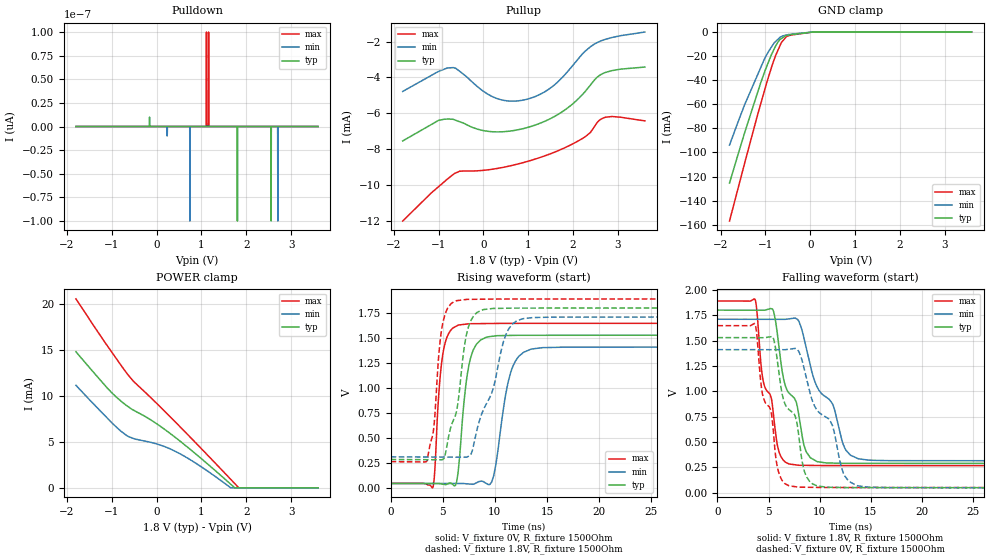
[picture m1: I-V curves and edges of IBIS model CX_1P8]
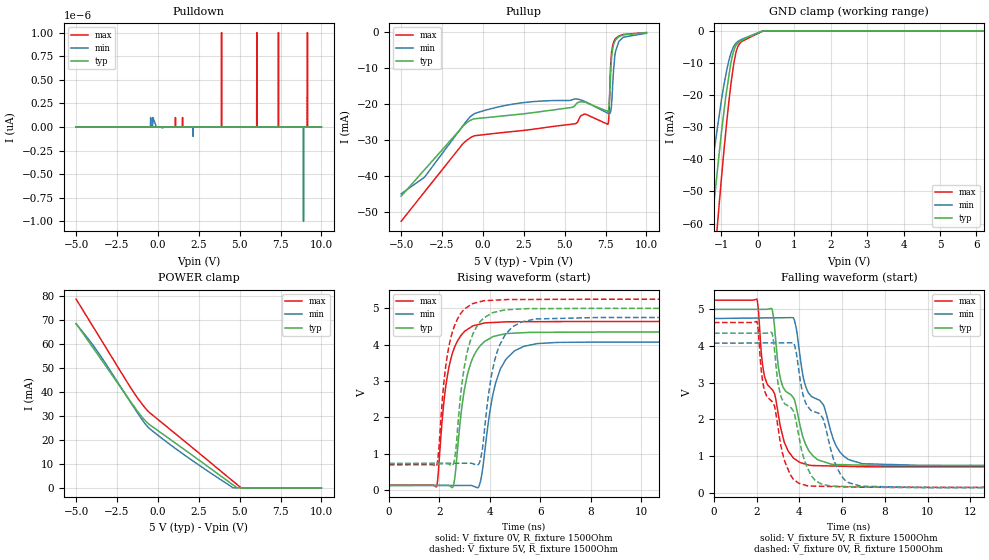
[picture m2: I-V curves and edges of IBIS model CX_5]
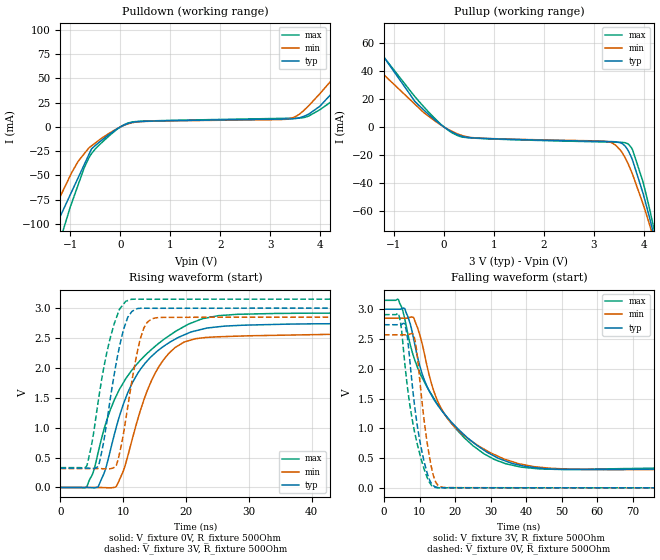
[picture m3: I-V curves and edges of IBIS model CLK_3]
| Texas Instruments Incorporated
| Smart Card Interface IC for 1 User Card + 3 SAMs
| Marketing part#   Voltage Range   Package-type   #pins/pkg drawing
| TCA5013ZAH   1.65V - 5.5V   nFBGA   48-pin ZAH
[IBIS Ver]   4.1
[File name]   tca5013.ibs
[File Rev]   1.0
[Date]   07/24/2014
[Source]   Model built from spectre simulations at:
   Texas Instruments Incorporated.
   Analog-eLab, HPA
   12500 TI Blvd
   Dallas, TX -75243
   For Support e-mail: elab_ibis@list.ti.com
[Notes]   Revision History
   Rev 1.0: 07/24/2014
   - Pullup and Pulldown is non-monotonic for many buffers
   - ccomp values are based on PVT settings:
   MIN: Low Voltage, High Temperature, Weak Process
   TYP: Nominal Voltage, Nominal Temperature, Nominal Process
   MAX: High Voltage, Low Temperature, Fast Process
   - C_comp although listed in numerical order of value are obtained from varying PVT conditions.
   For PVT conditions for each specific value, refer to the buffer description under respective [Model].
   IBIS model user is responsible for using appropriate C_comp to simulate for Signal Integrity.
[Disclaimer]  This model is designed as an aid for customers of Texas Instruments
 TI and its licensors and suppliers make no warranties, either expressed
 or implied, with respect to this  model, including the warranties of
 merchantability or fitness for a particular purpose.
 The model is provided solely on an "as is" basis. The entire risk as to
 its quality and performance is with the customer.
[Copyright] (C)Copyright 2014 Texas Instruments Incorporated.
   All rights reserved.
[Component]   TCA5013ZAH
[Manufacturer]  Texas Instruments Incorporated
[Package]   |48-pin nFBGA ZAH package
|   typ   min   max
R_pkg   0.005   0.005   0.005
L_pkg   0.2n   0.2n   0.2n
C_pkg   0.6p   0.6p   0.6p
[Pin]   signal_name   model_name   R_pin   L_pin   C_pin
A1   PRES   PRES   0.005   0.2nH   0.6pF
A2   GPIO4   GPIO   0.005   0.2nH   0.6pF
A4   GPIO3   GPIO   0.005   0.2nH   0.6pF
A5   GPIO2   GPIO   0.005   0.2nH   0.6pF
A6   GPIO1   GPIO   0.005   0.2nH   0.6pF
A8   VUP   NC   0.005   0.2nH   0.6pF
A9   LX   NC   0.005   0.2nH   0.6pF
B1   C8   CX   0.005   0.2nH   0.6pF
B2   A0   SCL   0.005   0.2nH   0.6pF
B3   INT   INT   0.005   0.2nH   0.6pF
B4   SHDN   PRES   0.005   0.2nH   0.6pF
B5   SCL   SCL   0.005   0.2nH   0.6pF
B6   SDA   SDA   0.005   0.2nH   0.6pF
B7   LDOCAP   NC   0.005   0.2nH   0.6pF
B8   TST4   NC   0.005   0.2nH   0.6pF
B9   GNDP   GND   0.005   0.2nH   0.6pF
C2   C4   CX   0.005   0.2nH   0.6pF
C8   VDD   POWER   0.005   0.2nH   0.6pF
D1   CLKUC   CLK   0.005   0.2nH   0.6pF
D2   TST3   NC   0.005   0.2nH   0.6pF
D8   GND   GND   0.005   0.2nH   0.6pF
D9   CLKIN1   CLKIN   0.005   0.2nH   0.6pF
E1   GNDUC   GND   0.005   0.2nH   0.6pF
E2   IOUC   IO   0.005   0.2nH   0.6pF
E8   IOMC1   IOMC   0.005   0.2nH   0.6pF
E9   GND   GND   0.005   0.2nH   0.6pF
F1   RSTUC   RST   0.005   0.2nH   0.6pF
F2   VCCUC   POWER   0.005   0.2nH   0.6pF
F8   IOMC2   IOMC   0.005   0.2nH   0.6pF
F9   CLKIN2   CLKIN   0.005   0.2nH   0.6pF
G2   TST2   NC   0.005   0.2nH   0.6pF
G8   VDDI   POWER   0.005   0.2nH   0.6pF
H1   RSTS3   RST   0.005   0.2nH   0.6pF
H2   IOS3   IO   0.005   0.2nH   0.6pF
H3   GNDS   GND   0.005   0.2nH   0.6pF
H4   TST1   NC   0.005   0.2nH   0.6pF
H5   IOS2   IO   0.005   0.2nH   0.6pF
H6   GNDS   GND   0.005   0.2nH   0.6pF
H7   GNDS   GND   0.005   0.2nH   0.6pF
H8   IOS1   IO   0.005   0.2nH   0.6pF
H9   VCCS1   POWER   0.005   0.2nH   0.6pF
J1   CLKS3   CLK   0.005   0.2nH   0.6pF
J2   VCCS3   POWER   0.005   0.2nH   0.6pF
J4   RSTS2   RST   0.005   0.2nH   0.6pF
J5   CLKS2   CLK   0.005   0.2nH   0.6pF
J6   VCCS2   POWER   0.005   0.2nH   0.6pF
J8   RSTS1   RST   0.005   0.2nH   0.6pF
J9   CLKS1   CLK   0.005   0.2nH   0.6pF
[Model Selector] CLK
CLK_1P8   CLK OUTPUT 1.8V
CLK_3   CLK OUTPUT 3V
CLK_5   CLK OUTPUT 5V
[Model Selector] CLKIN
CLKIN_1P8   CLKIN INPUT 1.8V
CLKIN_2P5   CLKIN INPUT 2.5V
CLKIN_3P3   CLKIN INPUT 3.3V
[Model Selector] RST
RST_1P8   RST OUTPUT 1.8V
RST_3   RST OUTPUT 3V
RST_5   RST OUTPUT 5V
[Model Selector] IO
IO_1P8   IO OUTPUT 1.8V
IO_3   IO OUTPUT 3V
IO_5   IO OUTPUT 5V
[Model Selector] IOMC
IOMC_1P8   IOMC OUTPUT 1.8V
IOMC_3   IOMC OUTPUT 3V
IOMC_5   IOMC OUTPUT 5V
[Model Selector] CX
CX_1P8   CX OUTPUT 1.8V
CX_3   CX OUTPUT 3V
CX_5   CX OUTPUT 5V
[Model Selector] SDA
SDA_1P8   SDA OPEN DRAIN I/O 1.8V
SDA_2P5   SDA OPEN DRAIN I/O 2.5V
SDA_3P3   SDA OPEN DRAIN I/O 3.3V
[Model Selector] GPIO
GPIO_1P8   GPIO OPEN DRAIN I/O 1.8V
GPIO_2P5   GPIO OPEN DRAIN I/O 2.5V
GPIO_3P3   GPIO OPEN DRAIN I/O 3.3V
[Model Selector] INT
INT_1P8   INT OPEN DRAIN OUTPUT 1.8V
INT_2P5   INT OPEN DRAIN OUTPUT 2.5V
INT_3P3   INT OPEN DRAIN OUTPUT 3.3V
[Model Selector] SCL
SCL_1P8   SCL INPUT 1.8V
SCL_2P5   SCL INPUT 2.5V
SCL_3P3   SCL INPUT 3.3V
[Model Selector] PRES
PRES_1P8   PRES INPUT 1.8V
PRES_2P5   PRES INPUT 2.5V
PRES_3P3   PRES INPUT 3.3V
| Models and submodels in the file (33): CX_1P8 (I/O), CX_3 (I/O), CX_5 (I/O), CLK_1P8 (Output), CLK_3 (Output), CLK_5 (Output), CLKIN_1P8 (Input), CLKIN_2P5 (Input), CLKIN_3P3 (Input), GPIO_1P8 (I/O_open_drain), GPIO_2P5 (I/O_open_drain), GPIO_3P3 (I/O_open_drain), INT_1P8 (Open_drain), INT_3P3 (Open_drain), INT_2P5 (Open_drain), IO_1P8 (I/O), IO_3 (I/O), IO_5 (I/O), IOMC_1P8 (I/O), IOMC_3 (I/O), IOMC_5 (I/O), PRES_1P8 (Input), PRES_2P5 (Input), PRES_3P3 (Input), RST_1P8 (Output), RST_3 (Output), RST_5 (Output), SCL_1P8 (Input), SCL_2P5 (Input), SCL_3P3 (Input), SDA_1P8 (I/O_open_drain), SDA_2P5 (I/O_open_drain), SDA_3P3 (I/O_open_drain)
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|   Model CX
[Model]   CX_1P8
Model_type   I/O
Polarity   Non-Inverting
Enable   Active-Low
Vinl = 0.72
Vinh = 1.08
Vmeas = 0.9
Vref = 1.8
Cref = 1pF
Rref = 1500
|   typ   min   max
C_comp   0.597p   0.445p   0.907p
|C_comp (ON state)   0.597p   0.445p   0.907p
|C_comp (OFF state)   0.592p   0.445p   0.907p
[Model spec]
|subparameter
Vinl   0.72   0.684   0.756
Vinh   1.08   1.026   1.134
[Voltage Range]   1.8   1.71   1.89
[Temperature Range]   27   125   -40
[Pullup Reference]   1.8   1.71   1.89
[Pulldown Reference]   0   0   0
[Power Clamp Reference]   1.8   1.71   1.89
[GND Clamp Reference]   0   0   0
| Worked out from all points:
|   slope of the pullup table from 0 to 0.27 V, typ, clamps not added: 3.81 kohm
|   GND clamp passes 1 mA (typ) near -0.17 V on its own axis
|   falling waveform, V_fixture 1.8V, R_fixture 1500Ohm: 20-80 % time 2.29ns typ, 3.31ns min, 1.65ns max; typ from 1.8 V to 0.289 V
|   rising waveform, V_fixture 0V, R_fixture 1500Ohm: 20-80 % time 876ps typ, 1.26ns min, 656ps max; typ from 0.05 V to 1.53 V
|   rising waveform, V_fixture 1.8V, R_fixture 1500Ohm: 20-80 % time 1.49ns typ, 2.43ns min, 743ps max; typ from 0.289 V to 1.8 V
|   falling waveform, V_fixture 0V, R_fixture 1500Ohm: 20-80 % time 2.27ns typ, 3.28ns min, 1.64ns max; typ from 1.53 V to 0.05 V
[Pulldown]
|   Voltage   I(typ)   I(min)   I(max)
-1.8V     0A         0A         0A
738mV     0A         0A         0A
743.4mV   0A         -100fA     0A
1.111V    0A         0A         100fA
1.802V    -100fA     0A         0A
1.807V    0A         0A         0A
2.547V    0A         0A         0A
2.552V    -100fA     0A         0A
2.698V    0A         0A         0A
2.704V    0A         -100fA     0A
2.709V    0A         0A         0A
3.6V      0A         0A         0A
[GND Clamp]
|   Voltage   I(typ)   I(min)   I(max)
-1.8V     -125.5mA   -93.9mA    -156.9mA
-1.465V   -83.92mA   -60.61mA   -109.3mA
-1.106V   -42.36mA   -29.69mA   -59.83mA
-995.4mV  -30.89mA   -20.6mA    -45.41mA
-844.2mV  -17.17mA   -11.26mA   -27.11mA
-774mV    -11.72mA   -7.931mA   -19.72mA
-725.4mV  -8.655mA   -6.195mA   -15.61mA
-644.4mV  -5.413mA   -3.754mA   -8.753mA
-531mV    -2.861mA   -2.501mA   -3.795mA
-423mV    -2.124mA   -1.831mA   -2.525mA
57.6mV    -11.54uA   -2.781uA   -1.994uA
3.6V      0A         0A         0A
[Pullup]
|   Voltage   I(typ)   I(min)   I(max)
-1.8V     -7.545mA   -4.782mA   -12.02mA
-995.4mV  -6.392mA   -3.659mA   -10.09mA
-671.4mV  -6.343mA   -3.451mA   -9.417mA
235.8mV   -7.037mA   -5.113mA   -9.112mA
565.2mV   -7.005mA   -5.317mA   -8.956mA
937.8mV   -6.827mA   -5.24mA    -8.722mA
1.397V    -6.417mA   -4.758mA   -8.355mA
1.796V    -5.852mA   -3.901mA   -7.948mA
2.266V    -4.796mA   -2.542mA   -7.32mA
2.525V    -4.014mA   -2.068mA   -6.556mA
2.698V    -3.745mA   -1.89mA    -6.242mA
3.6V      -3.421mA   -1.466mA   -6.428mA
[POWER Clamp]
|   Voltage   I(typ)   I(min)   I(max)
-1.8V     14.79mA    11.15mA    20.54mA
-1.106V   10.88mA    7.607mA    15.49mA
-806.4mV  9.478mA    6.196mA    13.41mA
-671.4mV  8.948mA    5.697mA    12.5mA
-487.8mV  8.37mA     5.314mA    11.45mA
9mV       6.94mA     4.761mA    9.145mA
370.8mV   5.655mA    4.077mA    7.389mA
916.2mV   3.506mA    2.542mA    4.669mA
1.651V    400.1uA    3.806uA    933uA
1.742V    472.3nA    0A         461.4uA
1.829V    0A         0A         16.54uA
3.6V      0A         0A         0A
[Ramp]
R_load = 1500
|   typ   min   max
dV/dt_r   0.887602/8.76301e-10   0.816767/1.2525e-09   0.957567/6.56016e-10
dV/dt_f   0.906661/2.28507e-09   0.836809/3.30284e-09   0.973581/1.65071e-09
[Falling Waveform]
V_fixture = 1.8V
V_fixture_min = 1.71V
V_fixture_max = 1.89V
R_fixture = 1500Ohm
C_fixture = 0F
|   Time   V(typ)   V(min)   V(max)
0s        1.8V       1.71V      1.89V
3.691ns   1.799V     1.71V      1.903V
4.406ns   1.799V     1.71V      1.144V
5.447ns   1.8V       1.709V     800.5mV
6.032ns   1.43V      1.709V     402.2mV
7.004ns   983.1mV    1.714V     285mV
7.984ns   752.5mV    1.687V     271.8mV
9.087ns   346.5mV    1.257V     270.5mV
13.75ns   290.7mV    337.8mV    268.7mV
49.9ns    288.9mV    315.3mV    267.4mV
[Rising Waveform]
V_fixture = 0V
V_fixture_min = 0V
V_fixture_max = 0V
R_fixture = 1500Ohm
C_fixture = 0F
|   Time   V(typ)   V(min)   V(max)
0s        49.9mV     49.46mV    51.37mV
4.08ns    50.23mV    49.68mV    18.4mV
4.995ns   43.34mV    49.73mV    1.33V
6.487ns   171.8mV    49.81mV    1.628V
7.524ns   1.234V     44.82mV    1.642V
9.209ns   1.509V     48.67mV    1.644V
9.895ns   1.519V     129.5mV    1.645V
11.51ns   1.526V     1.154V     1.646V
13.44ns   1.527V     1.387V     1.646V
49.9ns    1.529V     1.411V     1.647V
[Rising Waveform]
V_fixture = 1.8V
V_fixture_min = 1.71V
V_fixture_max = 1.89V
R_fixture = 1500Ohm
C_fixture = 0F
|   Time   V(typ)   V(min)   V(max)
0s        288.9mV    315.3mV    267.3mV
3.498ns   287mV      313.7mV    277.8mV
4.132ns   286.6mV    313.5mV    596.9mV
4.944ns   287.8mV    313.1mV    1.616V
6.301ns   760.3mV    312.5mV    1.871V
7.175ns   1.479V     312.1mV    1.883V
7.956ns   1.719V     429.7mV    1.886V
11.04ns   1.796V     1.527V     1.888V
12.58ns   1.798V     1.689V     1.888V
49.9ns    1.8V       1.71V      1.89V
[Falling Waveform]
|Gnd
V_fixture = 0V
V_fixture_min = 0V
V_fixture_max = 0V
R_fixture = 1500Ohm
C_fixture = 0F
|   Time   V(typ)   V(min)   V(max)
0s        1.529V     1.411V     1.647V
3.691ns   1.528V     1.41V      1.661V
4.406ns   1.528V     1.41V      973.8mV
5.447ns   1.53V      1.41V      637.3mV
5.956ns   1.232V     1.41V      214.7mV
7.004ns   820mV      1.415V     69.52mV
7.984ns   543.2mV    1.389V     56.13mV
9.019ns   113.7mV    1.001V     54.77mV
13.63ns   51.62mV    72.17mV    52.81mV
49.9ns    49.9mV     49.46mV    51.37mV
[Model]   CX_5
Model_type   I/O
Polarity   Non-Inverting
Enable   Active-Low
Vinl = 2
Vinh = 3
Vmeas = 2.5
Vref = 5
Cref = 1pF
Rref = 1500
|   typ   min   max
|   typ   min   max
C_comp   0.937p   0.723p   1.081p
|C_comp (ON state)   0.950p   0.730p   1.090p
|C_comp (OFF state)   0.937p   0.723p   1.081p
[Model spec]
|subparameter
Vinl   2.0   1.9   2.1
Vinh   3.0   2.85   3.15
[Voltage Range]   5   4.75   5.25
[Temperature Range]   27   125   -40
[Pullup Reference]   5   4.75   5.25
[Pulldown Reference]   0   0   0
[Power Clamp Reference]   5   4.75   5.25
[GND Clamp Reference]   0   0   0
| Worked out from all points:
|   GND clamp passes 1 mA (typ) near -0.05 V on its own axis
|   falling waveform, V_fixture 5V, R_fixture 1500Ohm: 20-80 % time 1.24ns typ, 1.56ns min, 1.04ns max; typ from 5 V to 0.725 V
|   rising waveform, V_fixture 0V, R_fixture 1500Ohm: 20-80 % time 550ps typ, 617ps min, 493ps max; typ from 0.132 V to 4.35 V
|   rising waveform, V_fixture 5V, R_fixture 1500Ohm: 20-80 % time 539ps typ, 596ps min, 486ps max; typ from 0.725 V to 5 V
|   falling waveform, V_fixture 0V, R_fixture 1500Ohm: 20-80 % time 1.29ns typ, 1.61ns min, 1.07ns max; typ from 4.35 V to 0.132 V
[Pulldown]
|   Voltage   I(typ)   I(min)   I(max)
-5V       0A         0A         0A
3.88V     0A         0A         0A
3.895V    0A         0A         1pA
3.91V     0A         0A         0A
6.04V     0A         0A         0A
6.055V    0A         0A         1pA
6.07V     0A         0A         0A
7.375V    0A         0A         1pA
8.89V     0A         0A         0A
8.905V    0A         -1pA       0A
9.145V    0A         0A         1pA
10V       0A         0A         0A
[GND Clamp]
|   Voltage   I(typ)   I(min)   I(max)
-5V       -2.369A    -1.94A     -2.673A
-2.405V   -203.9mA   -160.8mA   -244.3mA
-1.205V   -54.28mA   -38.24mA   -73.88mA
-995mV    -31.76mA   -21.64mA   -46.02mA
-875mV    -20.5mA    -13.85mA   -31.48mA
-725mV    -9.458mA   -6.709mA   -15.86mA
-650mV    -6.128mA   -4.72mA    -9.891mA
-590mV    -4.508mA   -3.781mA   -6.49mA
-545mV    -3.908mA   -3.328mA   -4.894mA
-455mV    -3.039mA   -2.739mA   -3.493mA
145mV     -91.73uA   -1.815uA   -57.07uA
10V       0A         0A         0A
[Pullup]
|   Voltage   I(typ)   I(min)   I(max)
-5V       -45.57mA   -44.92mA   -52.52mA
-3.569V   -38.25mA   -40.32mA   -44.39mA
-500mV    -24.14mA   -22.71mA   -28.84mA
5.68V     -20.21mA   -18.66mA   -25.48mA
6.25V     -19.59mA   -19.38mA   -22.86mA
7.645V    -22.14mA   -22.64mA   -25.7mA
7.705V    -20.96mA   -22.74mA   -23.32mA
7.84V     -9.039mA   -21.39mA   -7.208mA
7.99V     -3.646mA   -10.63mA   -2.972mA
8.11V     -2.346mA   -5.507mA   -1.961mA
8.32V     -1.416mA   -2.689mA   -1.214mA
10V       -326.4uA   -476.2uA   -291.8uA
[POWER Clamp]
|   Voltage   I(typ)   I(min)   I(max)
-5V       68.6mA     68.49mA    78.81mA
-4.205V   60.85mA    61.75mA    69.99mA
-3.569V   54.65mA    55.74mA    62.94mA
-1.415V   33.6mA     33.08mA    39.2mA
-995mV    29.76mA    28.81mA    35.26mA
-605mV    26.96mA    25.4mA     32.05mA
265mV     22.63mA    20.58mA    27.1mA
1.6V      16.09mA    13.84mA    19.65mA
4.6V      1.234mA    20.62uA    2.752mA
4.84V     50.39uA    0A         1.415mA
5.08V     0A         0A         81.65uA
10V       0A         0A         0A
[Ramp]
R_load = 1500
|   typ   min   max
dV/dt_r   2.52974/5.48999e-10   2.36911/6.16516e-10   2.70067/4.91468e-10
dV/dt_f   2.56493/1.23862e-09   2.407/1.55282e-09   2.73096/1.0265e-09
[Falling Waveform]
V_fixture = 5V
V_fixture_min = 4.75V
V_fixture_max = 5.25V
R_fixture = 1500Ohm
C_fixture = 0F
|   Time   V(typ)   V(min)   V(max)
0s        5V         4.75V      5.25V
2.008ns   5V         4.763V     5.278V
2.326ns   4.999V     4.765V     3.295V
2.7ns     5.024V     4.767V     2.825V
3.111ns   3.112V     4.77V      1.8V
3.725ns   2.58V      4.76V      938.9mV
4.462ns   1.125V     2.692V     746.6mV
5.9ns     761.2mV    1.103V     718.3mV
6.975ns   746.6mV    785.1mV    703.7mV
49.9ns    725.1mV    738.3mV    698.4mV
[Rising Waveform]
V_fixture = 0V
V_fixture_min = 0V
V_fixture_max = 0V
R_fixture = 1500Ohm
C_fixture = 0F
|   Time   V(typ)   V(min)   V(max)
0s        132mV      126.7mV    138.7mV
1.884ns   135.2mV    128.8mV    86.73mV
2.217ns   135.8mV    129.2mV    2.643V
2.538ns   83.95mV    129.6mV    3.801V
3.077ns   3.061V     130.2mV    4.4V
3.556ns   3.907V     86.86mV    4.554V
3.795ns   4.088V     1.022V     4.595V
4.436ns   4.271V     3.353V     4.618V
5.911ns   4.337V     4.031V     4.631V
49.9ns    4.348V     4.075V     4.64V
[Rising Waveform]
V_fixture = 5V
V_fixture_min = 4.75V
V_fixture_max = 5.25V
R_fixture = 1500Ohm
C_fixture = 0F
|   Time   V(typ)   V(min)   V(max)
0s        724.8mV    737.9mV    697.8mV
1.884ns   727.4mV    739.5mV    655.7mV
2.231ns   727.8mV    739.8mV    3.275V
2.538ns   686.2mV    740.1mV    4.39V
3.077ns   3.702V     740.6mV    5.016V
3.556ns   4.571V     709.2mV    5.168V
3.763ns   4.734V     1.473V     5.205V
4.396ns   4.923V     3.993V     5.228V
5.821ns   4.989V     4.705V     5.242V
49.9ns    5V         4.75V      5.25V
[Falling Waveform]
|Gnd
V_fixture = 0V
V_fixture_min = 0V
V_fixture_max = 0V
R_fixture = 1500Ohm
C_fixture = 0F
|   Time   V(typ)   V(min)   V(max)
0s        4.348V     4.075V     4.64V
2.008ns   4.348V     4.081V     4.669V
2.326ns   4.348V     4.082V     2.889V
2.7ns     4.374V     4.084V     2.496V
3.111ns   2.675V     4.085V     1.352V
3.725ns   2.219V     4.087V     360.9mV
4.345ns   714.8mV    2.385V     187.2mV
5.976ns   165.7mV    443.2mV    157mV
6.903ns   153.7mV    172.4mV    144.8mV
49.9ns    132mV      126.7mV    138.6mV
[Model]   CLK_3
Model_type   Output
Polarity   Non-Inverting
Vmeas = 1.5
Vref = 3
Cref = 1pF
Rref = 500
|   typ   min   max
C_comp   0.819p   0.538p   1.031p
|C_comp (ON state)   0.835p   0.552p   1.076p
|C_comp (OFF state)   0.819p   0.538p   1.031p
[Voltage Range]   3   2.85   3.15
[Temperature Range]   27   125   -40
[Pullup Reference]   3   2.85   3.15
[Pulldown Reference]   0   0   0
[Power Clamp Reference]   3   2.85   3.15
[GND Clamp Reference]   0   0   0
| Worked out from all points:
|   slope of the pulldown table from 0 to 0.45 V, typ, clamps not added: 78.7 ohm
|   slope of the pullup table from 0 to 0.45 V, typ, clamps not added: 61.4 ohm
|   falling waveform, V_fixture 3V, R_fixture 500Ohm: 20-80 % time 14.7ns typ, 12.8ns min, 14.9ns max; typ from 3 V to 0.324 V
|   rising waveform, V_fixture 0V, R_fixture 500Ohm: 20-80 % time 6.75ns typ, 5.22ns min, 8.74ns max; typ from 0 V to 2.74 V
|   rising waveform, V_fixture 3V, R_fixture 500Ohm: 20-80 % time 2.61ns typ, 2.5ns min, 2.9ns max; typ from 0.324 V to 3 V
|   falling waveform, V_fixture 0V, R_fixture 500Ohm: 20-80 % time 3.71ns typ, 3.17ns min, 4.55ns max; typ from 2.74 V to 0 V
[Pulldown]
|   Voltage   I(typ)   I(min)   I(max)
-3V       -452.1mA   -315.1mA   -713.3mA
-1.821V   -186.7mA   -149.6mA   -226mA
-1.254V   -99.02mA   -77.41mA   -125.1mA
-1.218V   -93.77mA   -73.23mA   -118.6mA
-849mV    -52.77mA   -35.72mA   -60.19mA
-579mV    -22.76mA   -19.61mA   -27.61mA
78mV      2.047mA    1.772mA    2.357mA
3.309V    8.145mA    7.847mA    8.892mA
3.696V    11.49mA    18.12mA    9.93mA
4.317V    39.85mA    53.6mA     30.44mA
5.127V    92.21mA    104.6mA    85.48mA
6V        151.3mA    163.6mA    150.8mA
[Pullup]
|   Voltage   I(typ)   I(min)   I(max)
-3V       141.7mA    144.7mA    151.2mA
-2.037V   92.54mA    82.48mA    88.04mA
-1.32V    55.94mA    41.24mA    55.29mA
-579mV    18.12mA    16.17mA    21.53mA
285mV     -5.762mA   -5.138mA   -6.381mA
3.336V    -10.46mA   -10.92mA   -10.85mA
3.579V    -12.14mA   -19.05mA   -11.1mA
3.759V    -22.32mA   -32.42mA   -15.23mA
3.984V    -47.28mA   -54.9mA    -39.18mA
4.11V     -64.1mA    -69.11mA   -57.6mA
4.299V    -91.31mA   -91.85mA   -88.15mA
6V        -448.7mA   -327.3mA   -572.1mA
[Ramp]
R_load = 500
|   typ   min   max
dV/dt_r   1.64604/6.7473e-09   1.54392/5.21966e-09   1.74768/8.74906e-09
dV/dt_f   1.60583/1.46791e-08   1.52272/1.27651e-08   1.68602/1.49498e-08
[Falling Waveform]
V_fixture = 3V
V_fixture_min = 2.85V
V_fixture_max = 3.15V
R_fixture = 500Ohm
C_fixture = 0F
|   Time   V(typ)   V(min)   V(max)
0s        3V         2.85V      3.15V
4.113ns   3V         2.85V      3.157V
5.875ns   3.008V     2.85V      2.828V
8.325ns   2.509V     2.863V     2.207V
11.4ns    1.805V     2.245V     1.775V
13.85ns   1.508V     1.657V     1.523V
17.24ns   1.227V     1.22V      1.222V
31.11ns   530.5mV    557.1mV    475.2mV
47ns      317mV      327.5mV    311.9mV
99.9ns    323.6mV    312.1mV    340mV
[Rising Waveform]
V_fixture = 0V
V_fixture_min = 0V
V_fixture_max = 0V
R_fixture = 500Ohm
C_fixture = 0F
|   Time   V(typ)   V(min)   V(max)
0s        87.73nV    485.2nV    71.04nV
4.201ns   137.7uV    116uV      14.7mV
6.013ns   11.51mV    165.8uV    587.9mV
8.907ns   1.013V     20.6mV     1.535V
11.4ns    1.739V     793mV      1.965V
13.31ns   2.055V     1.472V     2.19V
15.7ns    2.303V     2.025V     2.415V
18.26ns   2.48V      2.341V     2.607V
22.59ns   2.648V     2.502V     2.822V
99.9ns    2.743V     2.573V     2.913V
[Rising Waveform]
V_fixture = 3V
V_fixture_min = 2.85V
V_fixture_max = 3.15V
R_fixture = 500Ohm
C_fixture = 0F
|   Time   V(typ)   V(min)   V(max)
0s        323.6mV    315.5mV    331.9mV
4.153ns   323.8mV    315.7mV    356mV
6.013ns   358.6mV    315.8mV    1.438V
7.432ns   1.129V     310.7mV    2.28V
8.907ns   2.094V     372.6mV    2.839V
10.03ns   2.635V     893.5mV    3.064V
11.26ns   2.926V     1.697V     3.147V
13.31ns   2.999V     2.673V     3.149V
15.07ns   2.998V     2.836V     3.148V
99.9ns    3V         2.85V      3.15V
[Falling Waveform]
|Gnd
V_fixture = 0V
V_fixture_min = 0V
V_fixture_max = 0V
R_fixture = 500Ohm
C_fixture = 0F
|   Time   V(typ)   V(min)   V(max)
0s        2.74V      2.57V      2.909V
4.153ns   2.74V      2.57V      2.912V
4.86ns    2.742V     2.57V      2.691V
6.212ns   2.659V     2.57V      1.889V
8.399ns   1.488V     2.561V     1.002V
9.169ns   1.131V     2.315V     786.9mV
11.4ns    413.7mV    1.086V     299.1mV
14.35ns   17.01mV    127.8mV    5.957mV
17.24ns   510.3uV    4.588mV    242.5uV
99.9ns    67.36uV    114.5uV    36.16uV
